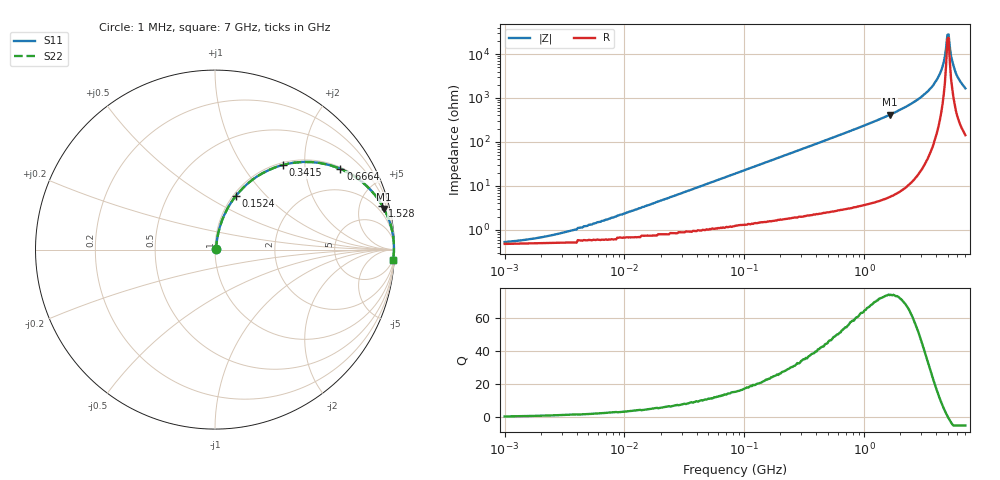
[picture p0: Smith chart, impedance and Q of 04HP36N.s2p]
# MHz S MA R 50
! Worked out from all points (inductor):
!   385 points, 1 MHz to 7 GHz, reference 50 ohm
!   read as one part in series: L = 36 nH near 8.151 MHz
!   highest Q = 74.2 at 1.638 GHz (marker M1), where L = 40.2 nH
!   self-resonance near 4.953 GHz
!   S11 on the Smith chart (normalised r, x): 1 MHz: 1.01, +0.00; 152.4 MHz: 1.03, +0.69; 341.5 MHz: 1.04, +1.55; 666.4 MHz: 1.06, +3.07; 1.528 GHz: 1.11, +7.62; 7 GHz: 4, -33
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1  0.005049 26.4  0.995 -0.1  0.995 -0.1  0.005049 26.4
1.952  0.006573 41.7  0.995 -0.3  0.995 -0.3  0.006573 41.7
4.374  0.011 60.1  0.994 -0.6  0.994 -0.6  0.011 60.1
19.575  0.045 77.5  0.991 -2.5  0.991 -2.5  0.045 77.5
85.617  0.188 75.5  0.97 -10.8  0.97 -10.8  0.188 75.5
152.368  0.322 68.7  0.933 -18.8  0.933 -18.8  0.322 68.7
341.475  0.605 51.2  0.78 -37.2  0.78 -37.2  0.605 51.2
365.931  0.632 49.3  0.759 -39.2  0.759 -39.2  0.632 49.3
666.414  0.831 32.8  0.541 -56.2  0.541 -56.2  0.831 32.8
1528.346  0.964 14.7  0.253 -74.6  0.253 -74.6  0.964 14.7
1637.803  0.969 13.5  0.234 -75.7  0.234 -75.7  0.969 13.5
2719.905  0.991 6.5  0.114 -82.4  0.114 -82.4  0.991 6.5
3756.121  0.996 3.0  0.052 -84.6  0.052 -84.6  0.996 3.0
4215.081  0.997 1.8  0.031 -83.7  0.031 -83.7  0.997 1.8
4516.955  0.997 1.1  0.019 -80.8  0.019 -80.8  0.997 1.1
4730.122  0.997 0.6  0.011 -74.3  0.011 -74.3  0.997 0.6
4840.449  0.997 0.4  0.006843 -65.0  0.006843 -65.0  0.997 0.4
4953.349  0.997 0.1  0.003657 -36.2  0.003657 -36.2  0.997 0.1
5068.882  0.997 -0.1  0.003578 31.6  0.003578 31.6  0.997 -0.1
5308.095  0.997 -0.6  0.011 71.4  0.011 71.4  0.997 -0.6
5820.923  0.996 -1.5  0.027 80.4  0.027 80.4  0.996 -1.5
7000  0.993 -3.4  0.06 81.7  0.06 81.7  0.993 -3.4
